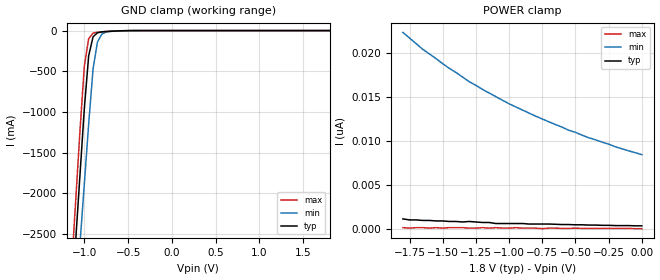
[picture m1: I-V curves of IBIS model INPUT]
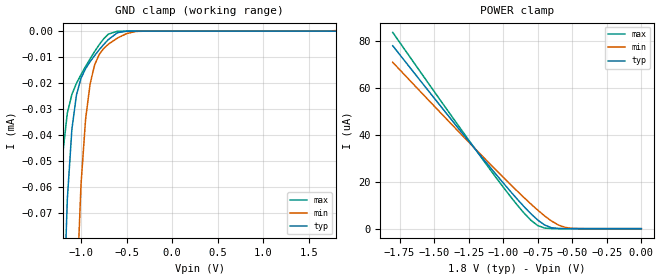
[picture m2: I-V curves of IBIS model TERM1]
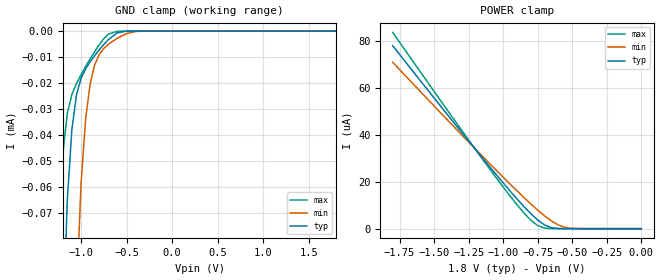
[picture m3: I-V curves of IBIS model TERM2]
|   DIODES INCORPORATED
|   IBIS Model of PI2SSD3212
|   Product Family: 2SSD
|   TFBGA (NC) Package
[IBIS Ver] 4.0
[Comment char] |_char
[File Name] pi2ssd3212_nc_18v.ibs
[File Rev] 1.0
[Source] File originated at Diodes Incorporated.
[Date] 04/22/19
[Disclaimer] (C) Copyright DIODES INCORPORATED
   All rights reserved
  Diodes Incorporated hereby grants the user of
  this IBIS model a non-exclusive, nontransferable license to
  use this IBIS model under the following terms.
  This IBIS model is provided on an "AS IS" basis and Diodes
  makes absolutely no warranty with respect to the information
  contained herein. DIODES DISCLAIMS AND CUSTOMER WAIVES ALL
  WARRANTIES, EXPRESSED OR IMPLIED, INCLUDING WARRANTIES OF
  MERCHANTABILITY OR FITNESS FOR A PARTICULAR PURPOSE. The
  entire risk as to quality and performance is with the customer.
  Accordingly, in no event shall the company be liable for any
  damages, whether in contract or tort, including any lost
  profits or other incidental, consequential, exemplary, or
  punitive damages arising out of the use or application of the
  IBIS model provided in this package. Further, Diodes reserves
  the right to make changes without notice to any product herein
  to improve reliability, function, or design. Diodes does not
  convey any license under patent rights or any other intellectual
  property rights, including those of third parties.
  The user is granted this license only to use the IBIS model
  and is not granted rights to sell, load, rent, lease or license
  the IBIS model in whole or in part, or in modified form to anyone
  other than user. User may modify the IBIS model to suit its specific
  application but rights to derivative works and such modifications
  shall belong to Diodes.
  Diodes is not obligated to provide maintenance or support
  for the licensed IBIS model.
  Contact Diodes at ATTN: APPLICATION ENGINEERING / IBIS MODELS
  1545 Barber Lane Milpitas, CA 95035 USA.
[Component] PI2SSD3212
[Manufacturer] Diodes Incorporated.
[Package]
| variable   typ   min   max
R_pkg   0.03740ohm   0.03260ohm   0.04220ohm
L_pkg   1.70900nH   1.57900nH   1.83900nH
C_pkg   0.87580pF   0.67460pF   1.07700pF
[Pin]   signal_name   model_name   R_pin   L_pin   C_pin
A1   B9   TERM2   0.04220   1.83900nH   1.07700pF
A2   B8   TERM2   0.03980   1.77400nH   0.97640pF
A3   B7   TERM2   0.03740   1.70900nH   0.87580pF
A4   C7   TERM2   0.03500   1.64400nH   0.77520pF
A5   C6   TERM2   0.03500   1.64400nH   0.77520pF
A6   B6   TERM2   0.03740   1.70900nH   0.87580pF
A7   B5   TERM2   0.03980   1.77400nH   0.97640pF
A8   B4   TERM2   0.04220   1.83900nH   1.07700pF
B1   B10   TERM2   0.03980   1.77400nH   0.97640pF
B2   C9   TERM2   0.03740   1.70900nH   0.87580pF
B3   C8   TERM2   0.03500   1.64400nH   0.77520pF
B4   GND   GND   0.03260   1.57900nH   0.67460pF
B5   VDD   POWER   0.03260   1.57900nH   0.67460pF
B6   C5   TERM2   0.03500   1.64400nH   0.77520pF
B7   C4   TERM2   0.03740   1.70900nH   0.87580pF
B8   B3   TERM2   0.03980   1.77400nH   0.97640pF
C1   B11   TERM2   0.03740   1.70900nH   0.87580pF
C2   C10   TERM2   0.03500   1.64400nH   0.77520pF
C7   C3   TERM2   0.03500   1.64400nH   0.77520pF
C8   B2   TERM2   0.03740   1.70900nH   0.87580pF
D1   C11   TERM2   0.03500   1.64400nH   0.77520pF
D2   EN   INPUT   0.03260   1.57900nH   0.67460pF
D7   SEL   INPUT   0.03260   1.57900nH   0.67460pF
D8   C2   TERM2   0.03500   1.64400nH   0.77520pF
E1   B12   TERM2   0.03500   1.64400nH   0.77520pF
E2   C12   TERM2   0.03260   1.57900nH   0.67460pF
E7   C1   TERM2   0.03260   1.57900nH   0.67460pF
E8   B1   TERM2   0.03500   1.64400nH   0.77520pF
F1   B13   TERM2   0.03740   1.70900nH   0.87580pF
F2   C13   TERM2   0.03500   1.64400nH   0.77520pF
F7   C0   TERM2   0.03500   1.64400nH   0.77520pF
F8   B0   TERM2   0.03740   1.70900nH   0.87580pF
G1   A13   TERM1   0.03980   1.77400nH   0.97640pF
G2   A11   TERM1   0.03740   1.70900nH   0.87580pF
G3   A9   TERM1   0.03500   1.64400nH   0.77520pF
G4   GND   GND   0.03260   1.57900nH   0.67460pF
G5   VDD   POWER   0.03260   1.57900nH   0.67460pF
G6   A4   TERM1   0.03500   1.64400nH   0.77520pF
G7   A2   TERM1   0.03740   1.70900nH   0.87580pF
G8   A0   TERM1   0.03980   1.77400nH   0.97640pF
H1   A12   TERM1   0.04220   1.83900nH   1.07700pF
H2   A10   TERM1   0.03980   1.77400nH   0.97640pF
H3   A8   TERM1   0.03740   1.70900nH   0.87580pF
H4   A7   TERM1   0.03500   1.64400nH   0.77520pF
H5   A6   TERM1   0.03500   1.64400nH   0.77520pF
H6   A5   TERM1   0.03740   1.70900nH   0.87580pF
H7   A3   TERM1   0.03980   1.77400nH   0.97640pF
H8   A1   TERM1   0.04220   1.83900nH   1.07700pF
[Series Switch Groups]
On 1 /
Off 2 /
[Series Pin Mapping]   pin_2   model_name  function_table_group
G8   F8   SWITCH1   1
H8   E8   SWITCH1   1
G7   C8   SWITCH1   1
H7   B8   SWITCH1   1
G6   A8   SWITCH1   1
H6   A7   SWITCH1   1
H5   A6   SWITCH1   1
H4   A3   SWITCH1   1
H3   A2   SWITCH1   1
G3   A1   SWITCH1   1
H2   B1   SWITCH1   1
G2   C1   SWITCH1   1
H1   E1   SWITCH1   1
G1   F1   SWITCH1   1
G8   F7   SWITCH1   2
H8   E7   SWITCH1   2
G7   D8   SWITCH1   2
H7   C7   SWITCH1   2
G6   B7   SWITCH1   2
H6   B6   SWITCH1   2
H5   A5   SWITCH1   2
H4   A4   SWITCH1   2
H3   B3   SWITCH1   2
G3   B2   SWITCH1   2
H2   C2   SWITCH1   2
G2   D1   SWITCH1   2
H1   E2   SWITCH1   2
G1   F2   SWITCH1   2
|   Model SWITCH1
[Model] SWITCH1
Model_type Series_switch
| variable   typ   min   max
C_comp   1.1408pF   0.7359pF   1.2215pF
[Voltage Range]   1.8000V   1.6200V   1.9800V
[GND Clamp Reference]   0.0000V   0.0000V   0.0000V
[POWER Clamp Reference]   1.8000V   1.6200V   1.9800V
[Temperature Range]   25   85   -10
[On]
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[OFF]
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| Models and submodels in the file (4): INPUT (Input), SWITCH1 (Series_switch), TERM1 (Terminator), TERM2 (Terminator)
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|   Model INPUT
[Model] INPUT
Model_type Input
Vinl = 800mV
Vinh = 2.0V
| variable   typ   min   max
C_comp   1.6846pF   1.6844pF   1.6848pF
[Voltage Range]   1.8000V   1.6200V   1.9800V
[GND Clamp Reference]   0.0000V   0.0000V   0.0000V
[POWER Clamp Reference]   1.8000V   1.6200V   1.9800V
[Temperature Range]   25   85   -10
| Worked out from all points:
|   GND clamp passes 1 mA (typ) near -0.51 V on its own axis
[GND Clamp]
| Voltage   I(typ)   I(min)   I(max)
-1.8V     -14.14A    -13.78A    -14.43A
-1.15V    -3.434A    -4.119A    -3.003A
-1.1V     -2.61A     -3.376A    -2.124A
-1.05V    -1.787A    -2.634A    -1.245A
-1V       -963.7mA   -1.891A    -439.9mA
-950mV    -309.6mA   -1.148A    -98.81mA
-900mV    -76.73mA   -470.7mA   -31.85mA
-850mV    -27.09mA   -141.9mA   -19.69mA
-800mV    -16.15mA   -42.85mA   -14.83mA
-750mV    -11.66mA   -17.83mA   -11.13mA
-400mV    -76.03uA   -213.9uA   -33.15uA
1.8V      378.3pA    9.284nA    87.31pA
[POWER Clamp]   |Note: Vtable = Vcc - Voutput
| Voltage   I(typ)   I(min)   I(max)
-1.8V     1.164nA    22.29nA    174.6pA
-1.75V    1.048nA    21.65nA    116.4pA
-1.65V    989.5pA    20.37nA    174.6pA
-1.45V    873.1pA    18.22nA    174.6pA
-1.3V     873.1pA    16.71nA    116.4pA
-1.15V    756.7pA    15.43nA    116.4pA
-1.1V     640.3pA    15.02nA    174.6pA
-1V       640.3pA    14.2nA     116.4pA
-800mV    582.1pA    12.81nA    116.4pA
-550mV    523.9pA    11.21nA    87.31pA
-200mV    407.5pA    9.342nA    87.31pA
0V        378.3pA    8.44nA     58.21pA
|   Model TERM1
[Model] TERM1
Model_type Terminator
| variable   typ   min   max
C_comp   1.2292pF   1.1332pF   1.7052pF
[Voltage Range]   1.8000V   1.6200V   1.9800V
[GND Clamp Reference]   0.0000V   0.0000V   0.0000V
[POWER Clamp Reference]   1.8000V   1.6200V   1.9800V
[Temperature Range]   25   85   -10
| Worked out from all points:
|   GND clamp passes 1 mA (typ) near -1.43 V on its own axis
[GND Clamp]
| Voltage   I(typ)   I(min)   I(max)
-1.8V     -19.99mA   -143.3mA   -6.049mA
-1.25V    -206.7uA   -655.5uA   -81.59uA
-1.2V     -116.4uA   -445uA     -47.23uA
-1.15V    -64.78uA   -286.8uA   -31.56uA
-1.1V     -37.79uA   -175.6uA   -24.36uA
-1.05V    -24.6uA    -103.1uA   -20.14uA
-950mV    -14.48uA   -34.03uA   -13.64uA
-900mV    -11.77uA   -20.3uA    -10.66uA
-800mV    -7.162uA   -8.979uA   -5.205uA
-700mV    -3.234uA   -5.048uA   -1.137uA
-400mV    -516.6pA   -116.9nA   -36.38pA
1.8V      87.31pA    227.1nA    87.31pA
[POWER Clamp]   |Note: Vtable = Vcc - Voutput
| Voltage   I(typ)   I(min)   I(max)
-1.8V     78.1uA     71.01uA    83.78uA
-1.4V     48.38uA    46.17uA    50.24uA
-1.1V     26.57uA    27.89uA    25.66uA
-900mV    12.71uA    16.13uA    10.2uA
-800mV    6.402uA    10.55uA    3.616uA
-750mV    3.672uA    7.912uA    1.307uA
-700mV    1.551uA    5.445uA    250.4nA
-650mV    401.2nA    3.258uA    31.37nA
-600mV    68.83nA    1.541uA    3.696nA
-550mV    10.33nA    515.7nA    465.7pA
-450mV    261.9pA    26.54nA    87.31pA
0V        87.31pA    29.1pA     58.21pA
|   Model TERM2
[Model] TERM2
Model_type Terminator
| variable   typ   min   max
C_comp   1.1332pF   0.5443pF   1.2217pF
[Voltage Range]   1.8000V   1.6200V   1.9800V
[GND Clamp Reference]   0.0000V   0.0000V   0.0000V
[POWER Clamp Reference]   1.8000V   1.6200V   1.9800V
[Temperature Range]   25   85   -10
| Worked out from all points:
|   GND clamp passes 1 mA (typ) near -1.43 V on its own axis
[GND Clamp]
| Voltage   I(typ)   I(min)   I(max)
-1.8V     -15.22mA   -92.46mA   -5.486mA
-1.25V    -205uA     -643.2uA   -81.34uA
-1.2V     -115.8uA   -438.2uA   -47.16uA
-1.15V    -64.59uA   -283.4uA   -31.54uA
-1.1V     -37.73uA   -174.1uA   -24.35uA
-1.05V    -24.58uA   -102.5uA   -20.13uA
-950mV    -14.48uA   -33.95uA   -13.63uA
-900mV    -11.77uA   -20.28uA   -10.65uA
-800mV    -7.16uA    -8.974uA   -5.204uA
-700mV    -3.233uA   -5.046uA   -1.137uA
-400mV    -523.9pA   -116.8nA   -14.55pA
1.8V      0A         227.1nA    0A
[POWER Clamp]   |Note: Vtable = Vcc - Voutput
| Voltage   I(typ)   I(min)   I(max)
-1.8V     78.1uA     71.01uA    83.78uA
-1.4V     48.38uA    46.17uA    50.24uA
-1.1V     26.57uA    27.89uA    25.66uA
-900mV    12.71uA    16.13uA    10.2uA
-800mV    6.402uA    10.55uA    3.616uA
-750mV    3.672uA    7.912uA    1.307uA
-700mV    1.551uA    5.445uA    250.4nA
-650mV    401.2nA    3.258uA    31.37nA
-600mV    68.83nA    1.541uA    3.696nA
-550mV    10.33nA    515.7nA    465.7pA
-450mV    261.9pA    26.54nA    87.31pA
0V        87.31pA    29.1pA     58.21pA
